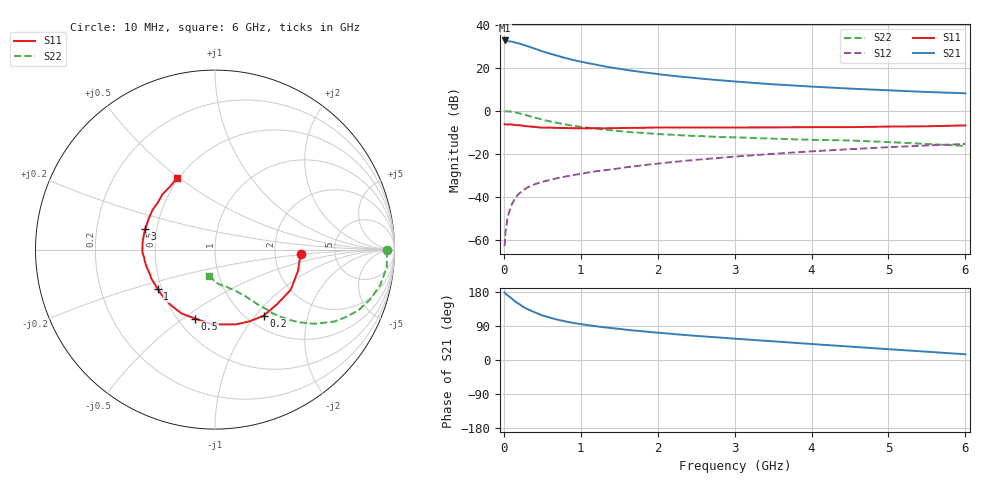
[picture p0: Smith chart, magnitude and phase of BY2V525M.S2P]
! SIEMENS Small Signal Semiconductors
! BFY420
! Si NPN RF SIEGET Grounded Emitter Transistor in MICRO-X
! VCE = 2.5 V  IC = 25 mA
! Common Emitter S-Parameters:  October  1996
# GHz  S  MA  R  50
!  f  S11  S21  S12  S22
! GHz  MAG  ANG  MAG  ANG  MAG  ANG  MAG  ANG
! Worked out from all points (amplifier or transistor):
!   36 points, 10 MHz to 6 GHz, reference 50 ohm
!   highest |S21| = 32.7 dB at 10 MHz (marker M1)
!   |S21| within 3 dB of that: start of sweep to 334.9 MHz
!   unconditionally stable (mu >= 1): 1.765 GHz to end of sweep
!   at 250 MHz: K = 0.33, MSG = 33.9 dB, |S12| = -37.1 dB
!   at 1.4 GHz: K = 0.95, MSG = 23.7 dB, |S12| = -27.4 dB
!   at 6 GHz: K = 1.07, MAG = 10.2 dB, |S12| = -15.5 dB
!   S11 on the Smith chart (normalised r, x): 10 MHz: 2.84, -0.19; 200 MHz: 1.19, -1.10; 500 MHz: 0.61, -0.56; 1 GHz: 0.48, -0.25; 3 GHz: 0.43, +0.12; 6 GHz: 0.49, +0.49
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0.01  0.4807 -3.1  42.95 178.4  0.0007 122.4  0.956 -0.3
0.02  0.4755 -6.1  42.65 175.4  0.0014 89.1  0.9587 -1.7
0.05  0.4776 -14.3  41.38 170.5  0.0034 87.6  0.9619 -5.8
0.1  0.4776 -28.0  40.4 162.8  0.0064 82.2  0.9418 -12.1
0.15  0.4605 -41.1  38.42 154.0  0.0094 74.0  0.9073 -17.9
0.2  0.4572 -53.6  36.49 147.5  0.0118 71.2  0.8682 -22.9
0.25  0.4437 -64.4  34.15 140.6  0.0139 67.6  0.8199 -27.3
0.3  0.4324 -74.5  31.94 134.9  0.016 66.4  0.7764 -31.1
0.4  0.4171 -92.0  27.75 125.9  0.0193 62.8  0.6903 -36.8
0.5  0.4002 -106.1  23.98 117.6  0.022 61.0  0.6192 -40.8
0.6  0.4015 -117.3  21.16 111.7  0.0243 59.9  0.5619 -43.8
0.7  0.3958 -126.6  18.82 106.3  0.0269 60.6  0.5153 -46.1
0.8  0.394 -133.8  16.77 101.8  0.0292 58.7  0.4764 -48.0
1  0.3876 -145.4  13.81 94.7  0.0337 59.8  0.42 -50.2
1.1  0.3868 -151.0  12.69 91.8  0.0364 60.1  0.3976 -51.6
1.6  0.3952 -169.0  8.81 79.6  0.0483 60.2  0.3207 -56.1
2.2  0.4046 177.4  6.439 68.7  0.0637 58.3  0.274 -61.2
3  0.4051 163.6  4.764 56.3  0.085 54.0  0.239 -67.2
3.5  0.4076 155.5  4.099 49.3  0.0987 50.6  0.2225 -71.2
4.5  0.4125 140.6  3.252 35.4  0.1266 42.4  0.2016 -79.9
5.5  0.4319 125.0  2.715 21.9  0.1545 33.1  0.1674 -93.6
6  0.4521 118.1  2.533 15.0  0.1678 28.3  0.1504 -103.3
